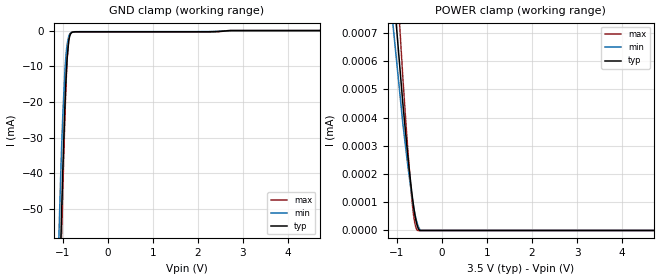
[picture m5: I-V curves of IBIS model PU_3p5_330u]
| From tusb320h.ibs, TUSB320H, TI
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|   Model
[Model]   PU_3p5_330u
Model_type   Input
Vinl = 1.05
Vinh = 2.45
|   typ   min   max
C_comp   1pF   1pF   1pF
[Voltage Range]   3.5   3.499   3.501
[Temperature Range]   27   105   -40
[Power Clamp Reference]   3.5   3.499   3.501
[GND Clamp Reference]   0   0   0
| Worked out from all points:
|   GND clamp passes 1 mA (typ) near -0.82 V on its own axis
[GND Clamp]
|   Voltage   I(typ)   I(min)   I(max)
-3.5V     -1.465A    -1.389A    -1.519A
-1.127V   -102.9mA   -77.81mA   -113.9mA
-1.043V   -61.2mA    -41.4mA    -69.12mA
-1.032V   -56.28mA   -37.33mA   -63.75mA
-1.022V   -51.45mA   -33.39mA   -58.46mA
-1.012V   -46.73mA   -29.62mA   -53.24mA
-990.5mV  -37.65mA   -22.65mA   -43.12mA
-948.5mV  -21.5mA    -11.48mA   -24.6mA
-906.5mV  -9.498mA   -4.724mA   -10.19mA
-864.5mV  -3.086mA   -1.732mA   -2.644mA
-801.5mV  -618.3uA   -520.7uA   -503.5uA
7V        0A         0A         0A
[POWER Clamp]
|   Voltage   I(typ)   I(min)   I(max)
-3.5V     5.553uA    1.275mA    7.545uA
-3.059V   4.68uA     3.893uA    6.352uA
-864.5mV  452.9nA    381.7nA    545.2nA
-749mV    259.8nA    225.7nA    278.8nA
-707mV    195.2nA    173.8nA    191.3nA
-665mV    135.6nA    125.9nA    113.7nA
-633.5mV  95.61nA    93.52nA    65.69nA
-602mV    61.17nA    64.95nA    30.2nA
-570.5mV  33.83nA    41.04nA    8.968nA
-539mV    14.62nA    22.46nA    0A
-476mV    0A         0A         0A
7V        0A         0A         0A
